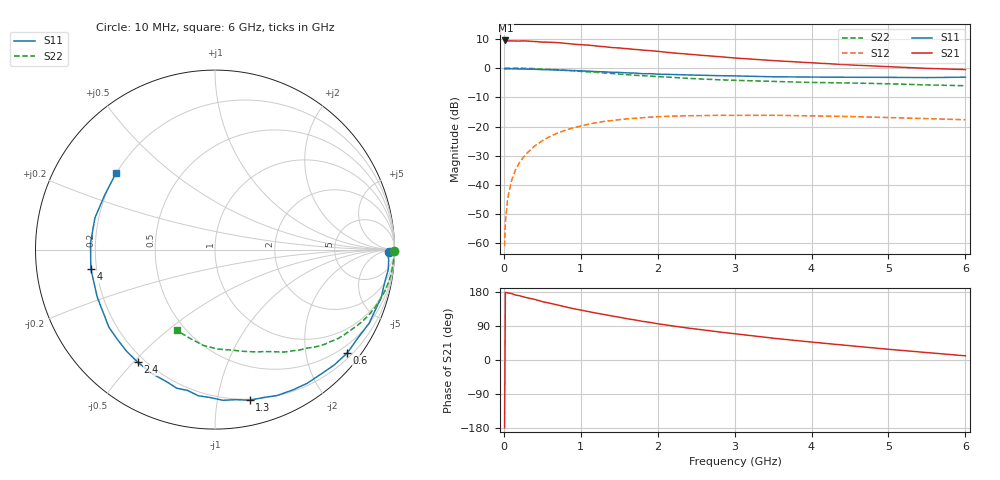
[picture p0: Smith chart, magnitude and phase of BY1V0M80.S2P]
! SIEMENS Small Signal Semiconductors
! BFY420
! Si NPN RF SIEGET Grounded Emitter Transistor in MICRO-X
! VCE = 1 V  IC = 0.8 mA
! Common Emitter S-Parameters:  October  1996
# GHz  S  MA  R  50
!  f  S11  S21  S12  S22
! GHz  MAG  ANG  MAG  ANG  MAG  ANG  MAG  ANG
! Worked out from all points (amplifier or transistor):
!   36 points, 10 MHz to 6 GHz, reference 50 ohm
!   highest |S21| = 9.4 dB at 20 MHz (marker M1)
!   |S21| within 3 dB of that: start of sweep to 1.679 GHz
!   unconditionally stable (mu >= 1): 4.663 GHz to end of sweep
!   at 250 MHz: K = 0.04, MSG = 20.0 dB, |S12| = -30.7 dB
!   at 1.4 GHz: K = 0.22, MSG = 12.5 dB, |S12| = -18.0 dB
!   at 6 GHz: K = 1.34, MAG = 5.1 dB, |S12| = -17.7 dB
!   S11 on the Smith chart (normalised r, x): 10 MHz: 51, -22; 600 MHz: 0.31, -2.87; 1.3 GHz: 0.19, -1.24; 2.4 GHz: 0.17, -0.51; 4 GHz: 0.18, -0.08; 6 GHz: 0.20, +0.33
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0.01  0.9675 -0.8  2.957 -179.3  0.0009 102.1  0.9978 -0.4
0.02  0.9611 -1.3  2.958 178.7  0.0023 85.0  0.9963 -0.6
0.05  0.9694 -3.3  2.902 177.0  0.0059 89.5  0.998 -1.7
0.1  0.9716 -6.7  2.909 175.3  0.0118 86.4  0.9969 -3.5
0.15  0.9646 -9.6  2.897 171.6  0.0179 83.3  0.9928 -5.2
0.2  0.9619 -12.9  2.888 169.8  0.0238 82.9  0.9931 -6.8
0.3  0.9566 -19.1  2.892 164.3  0.0351 77.7  0.9859 -10.2
0.5  0.9362 -31.6  2.776 154.0  0.0571 69.9  0.9622 -16.7
0.6  0.9352 -38.0  2.76 149.8  0.0676 66.0  0.9477 -19.9
0.8  0.9108 -49.6  2.641 140.3  0.0863 58.2  0.9137 -25.9
1.1  0.8834 -67.0  2.461 127.8  0.1095 48.0  0.8596 -33.9
1.3  0.8614 -77.0  2.32 120.2  0.1219 41.8  0.8228 -38.5
1.6  0.8242 -92.1  2.141 109.0  0.1351 33.1  0.7693 -45.1
1.8  0.7993 -101.1  2.027 102.1  0.1413 28.4  0.7396 -48.6
2.2  0.7744 -117.3  1.809 89.8  0.1504 19.5  0.6908 -55.7
2.4  0.7608 -124.5  1.725 84.1  0.1527 16.1  0.6651 -58.9
2.8  0.7386 -137.6  1.564 74.0  0.1554 9.5  0.6289 -64.6
3.5  0.7077 -157.9  1.339 57.6  0.1556 0.5  0.59 -74.0
4  0.7002 -171.1  1.229 47.3  0.1519 -4.7  0.5664 -81.1
4.5  0.6944 176.9  1.13 37.7  0.1481 -9.2  0.5544 -88.4
5.5  0.6856 153.4  0.986 19.6  0.1364 -14.5  0.5138 -105.7
6  0.6969 142.4  0.94 11.0  0.1305 -15.2  0.498 -115.4
